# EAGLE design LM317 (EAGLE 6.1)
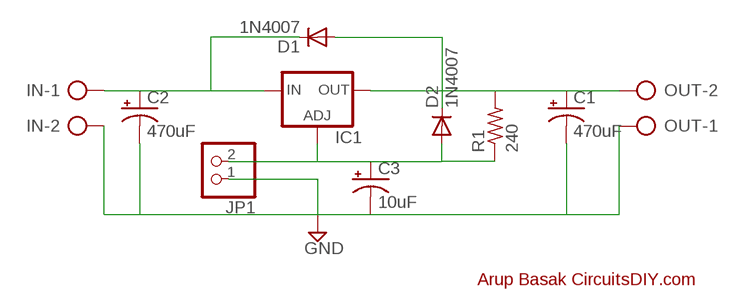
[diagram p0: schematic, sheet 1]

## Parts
C1  470uF  CPOL-USE3.5-8  [E3,5-8]
C2  470uF  CPOL-USE3.5-8  [E3,5-8]
C3  10uF  CPOL-USE2.5-5  [E2,5-5]
D1  1N4007  1N4004  [DO41-10]
D2  1N4007  1N4004  [DO41-10]
IC1  LM317TS  [317TS]
IN  AK500/2  [AK500/2]
JP1  PINHD-1X2  [1X02]
OUT  AK500/2  [AK500/2]
R1  240  R-US_0207/10  [0207/10]

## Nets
GND: C1.- C2.- C3.- IN.2 JP1.1 OUT.1
N$1: C2.+ D1.C IC1.3(IN) IN.1
N$2: C1.+ D1.A D2.C IC1.2(OUT) OUT.2 R1.2
N$3: C3.+ D2.A IC1.1(ADJ) JP1.2 R1.1

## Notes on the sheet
- Arup Basak CircuitsDIY.com

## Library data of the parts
C1-C3 = rcl:CPOL-US: POLARIZED CAPACITOR, American symbol
D1 D2 = diode:1N4004: DIODE
IC1 = v-reg:LM317TS: VOLTAGE REGULATOR
IN OUT = con-ptr500:AK500/2: CONNECTOR; OC_FARNELL: unknown; OC_NEWARK: unknown
JP1 = pinhead:PINHD-1X2: PIN HEADER
R1 = resistor:R-US_: RESISTOR, American symbol

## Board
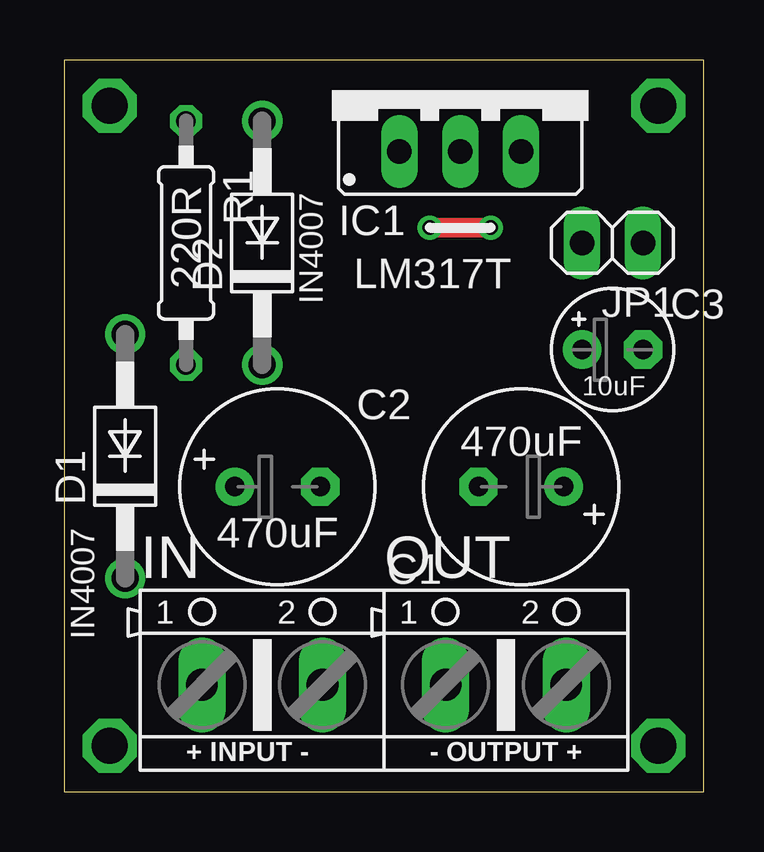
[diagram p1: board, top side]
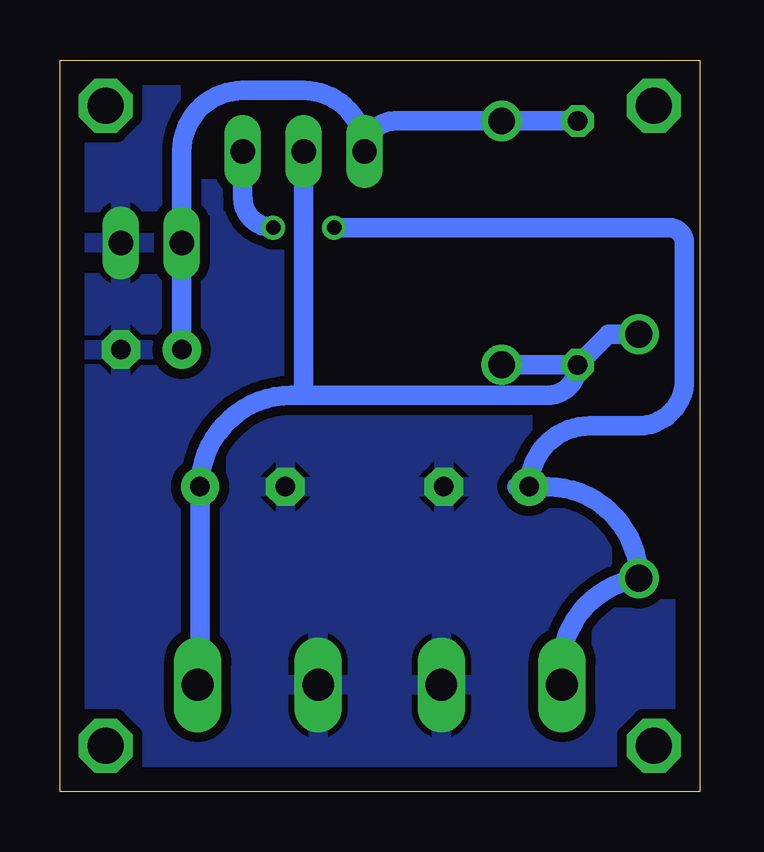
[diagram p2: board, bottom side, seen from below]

Size 26.67 x 30.48 mm. Coordinates in mm from the lower left corner, seen from the top.
Outline: 0,0 26.67,0 26.67,30.48 0,30.48 0,0
Copper layers (1*16): Top 0.035mm / dielectric 1.5mm / Bottom 0.035mm
Design rules: minimum track width 10mil, minimum drill 24mil, track to track 8mil, track to pad 8mil, pad to pad 8mil, via to via 8mil, smd to smd 8mil, copper to edge 40mil, drill to drill 8mil, minimum pad ring 10mil, minimum via ring 8mil, stop-mask expansion 4mil, vias tented up to drill 0mil, thermal gap 10mil

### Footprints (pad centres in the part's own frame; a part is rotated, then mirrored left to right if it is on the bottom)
E3,5-8 = drill 0.813 pad 1.6: + -1.778,0 | drill 0.813 pad 1.6 octagon: - 1.778,0
E2,5-5 = drill 0.813 pad 1.6: + -1.27,0 | drill 0.813 pad 1.6 octagon: - 1.27,0
DO41-10 = drill 1.118: A 5.08,0; C -5.08,0
317TS = drill 1.016 long: 1 -2.54,-2.54; 2 0,-2.54; 3 2.54,-2.54
AK500/2 = drill 1.321 long: 1 -2.515,0; 2 2.515,0
1X02 = drill 1.016 long: 1 -1.27,0; 2 1.27,0
0207/10 = drill 0.813 octagon: 1 -5.08,0; 2 5.08,0

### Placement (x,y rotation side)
C1  19.05,12.7 180 top
C2  8.89,12.7 0 top
C3  22.86,18.41 0 top
D1  2.54,13.97 90 top
D2  8.25,22.86 90 top
IC1  16.51,29.21 0 top
IN  8.25,4.45 0 top
JP1  22.86,22.86 180 top
OUT  18.41,4.45 0 top
R1  5.08,22.86 270 top

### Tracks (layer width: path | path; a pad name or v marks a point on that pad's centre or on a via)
GND
  pour Bottom (isolate 0.406): 0,30.48 26.67,30.48 26.67,0 0,0
N$1  (via drill 0.6)
  Top 0.813: v15.24,23.5 v17.78,23.5
  Bottom 0.813: IN.1 arc90 2.57,8.89 D1.C arc-90 6.35,12.7 C2.+ | C2.+ 7.62,12.7 | C2.+ arc90 4.57,15.24 2.54,15.24 arc-90 0.63,17.14 0.63,22.86 arc-90 1.27,23.5 v15.24,23.5 | v17.78,23.5 arc90 19.05,24.77 IC1.3
N$2
  Bottom 0.813: D1.A 3.81,19.05 R1.2 | OUT.2 20.83,4.55 C1.+ arc90 17.02,16.51 16.51,16.51 | 16.51,16.51 6.35,16.51 arc-90 R1.2 | R1.2 D2.C | IC1.2 16.51,16.51
N$3
  Bottom 0.813: R1.1 D2.A 12.7,27.94 arc-90 IC1.1 arc-90 16.51,29.21 19.05,29.21 arc-90 21.59,26.67 JP1.2 C3.+
N$4  (via drill 1.5)
  other vias: 1.91,1.91
N$5  (via drill 1.5)
  other vias: 24.77,1.91
N$6  (via drill 1.5)
  other vias: 24.77,28.57
N$7  (via drill 1.5)
  other vias: 1.91,28.57

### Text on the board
tPlace: 220R | LM317T | IN4007 | 10uF | 470uF | 470uF | IN4007 | + INPUT - | - OUTPUT +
